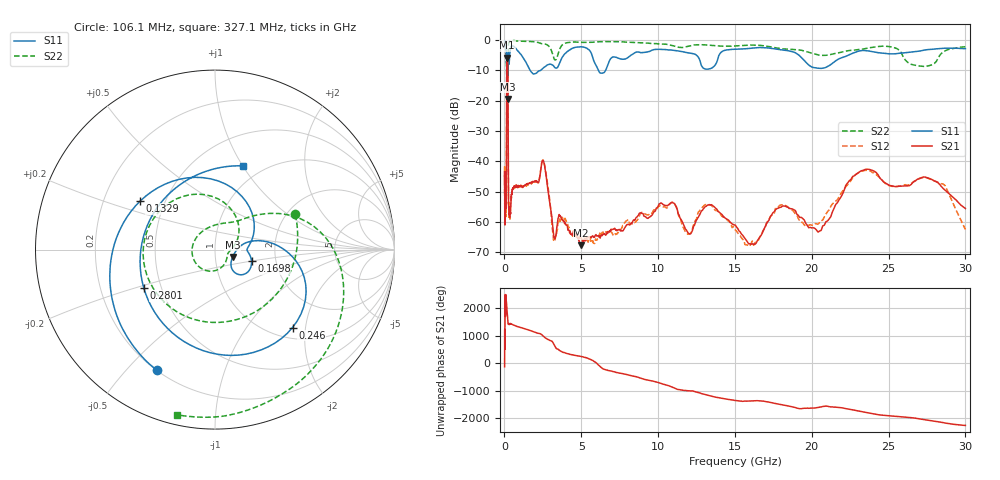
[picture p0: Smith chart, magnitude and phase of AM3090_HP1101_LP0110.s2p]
! Date/Time: Thu, Feb 28, 2019 2:07 PM
! Network Analyzer: Agilent Technologies E8364B Rev: A.07.50.67
! Sweep from 0.010 to 30.000 GHz, 1601 Points, Sweep Type: LOG
! Power Supply: 5.022 V, 0.002 A
# Hz S DB R 50
!freq MagS11 AngS11 MagS21 AngS21 MagS12 AngS12 MagS22 AngS22
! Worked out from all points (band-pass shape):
!   1601 points, 10 MHz to 30 GHz, reference 50 ohm
!   highest |S21| = -5.80 dB at 180.3 MHz (marker M1); lowest = -67.6 dB at 5.002 GHz (marker M2)
!   |S21| within 3 dB of the highest: 150.7 MHz to 216.3 MHz (65.66 MHz wide, 35.8 % of centre)
!   lowest |S11| = -19.5 dB at 203.4 MHz (marker M3), VSWR 1.24, Z = 60.7 - j5.03 ohm
!   |S11| at or under -10 dB: 144 MHz to 225.3 MHz (81.27 MHz wide, 44 % of centre); 1.669 GHz to 2.36 GHz (690.5 MHz wide, 34.3 % of centre); 6.11 GHz to 6.585 GHz (474.7 MHz wide, 7.48 % of centre)
!   |S22| runs from -22.5 to -0.2 dB; largest |S21 - S12| = 0.012
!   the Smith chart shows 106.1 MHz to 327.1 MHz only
!   S11 on the Smith chart (normalised r, x): 106.1 MHz: 0.20, -0.61; 132.9 MHz: 0.36, +0.26; 169.8 MHz: 1.49, -0.20; 246 MHz: 1.22, -1.70; 280.1 MHz: 0.40, -0.21; 327.1 MHz: 0.82, +1.00
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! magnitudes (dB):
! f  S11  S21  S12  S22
! 10 MHz  -0.3  -47.7  -41.6  -0.6
! 38.04 MHz  -0.4  -58.7  -58.4  -1.3
! 48.61 MHz  -0.5  -49.0  -48.2  -1.3
! 106.1 MHz  -2.5  -55.1  -53.6  -6.2
! 132.9 MHz  -6.1  -28.5  -28.4  -8.0
! 144.7 MHz  -10.3  -12.7  -12.6  -12.6
! 169.8 MHz  -13.4  -6.0  -5.9  -19.7
! 180.3 MHz  -13.1  -5.8  -5.8  -17.8
! 203.4 MHz  -19.5  -6.7  -6.7  -17.8
! 246 MHz  -4.3  -37.6  -37.9  -2.8
! 280.1 MHz  -6.9  -55.4  -54.2  -1.0
! 327.1 MHz  -6.2  -58.0  -56.5  -0.5
! 550.5 MHz  -2.0  -48.8  -49.3  -0.3
! 2.084 GHz  -10.9  -46.5  -46.8  -0.7
! 2.533 GHz  -9.2  -39.8  -39.6  -1.3
! 3.204 GHz  -8.6  -64.4  -66.0  -5.8
! 5.002 GHz  -2.3  -67.6  -65.4  -0.8
! 7.926 GHz  -6.1  -61.1  -59.6  -0.7
! 13.34 GHz  -9.5  -54.2  -54.3  -1.7
! 16.05 GHz  -2.7  -67.3  -67.1  -1.7
! 23.59 GHz  -3.6  -42.6  -42.9  -2.7
! 30 GHz  -2.9  -55.5  -62.4  -2.3
